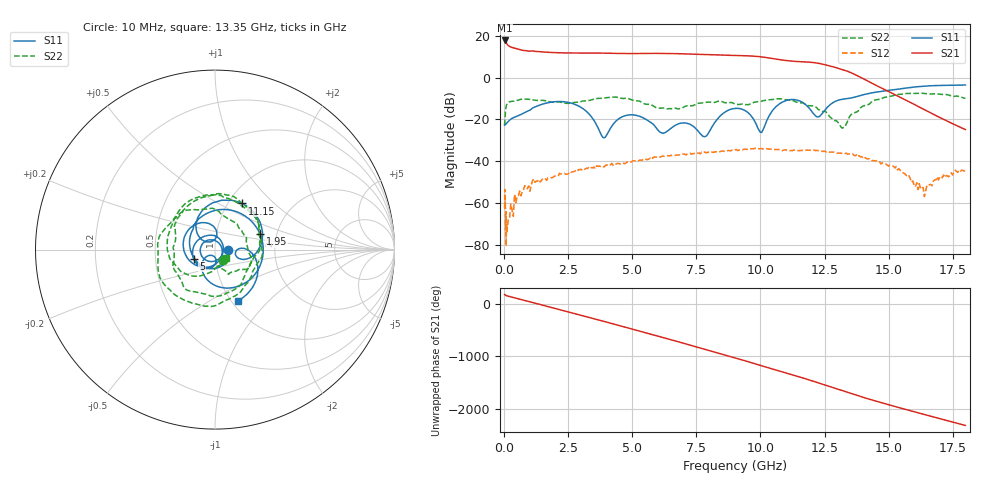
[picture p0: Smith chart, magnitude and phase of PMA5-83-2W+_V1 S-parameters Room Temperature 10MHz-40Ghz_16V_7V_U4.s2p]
!Mini-Circuits Laboratory
!S-Parameters
!Model: US-AMP-1
!Run / Lot / Date Code: N/A /  / N/A
!Fixture: ON TB-
!Network Analyzer: NFA N8975A;  Serial number: 74408
!Date: 12/1/2023 at 8:04:13 AM
!No.: Unit# 1 (#1)
!Tested with:
!Condition 5: Vdd = +16V; Vg2= +7V; Idd= 400mA
# Hz  S  dB  R  50
!Frequency  S11 dB  S11 Deg  S21 dB  S21 Deg  S12 dB  S12 Deg  S22 dB  S22 Deg
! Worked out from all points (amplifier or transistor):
!   368 points, 10 MHz to 18 GHz, reference 50 ohm
!   highest |S21| = 17.8 dB at 20 MHz (marker M1)
!   |S21| within 3 dB of that: start of sweep to 227.9 MHz
!   unconditionally stable (mu >= 1): start of sweep to end of sweep
!   at 2.7 GHz: K = 19.95, MAG = 12.4 dB, |S12| = -44.9 dB
!   at 8.85 GHz: K = 7.35, MAG = 11.2 dB, |S12| = -34.9 dB
!   at 18 GHz: K = 696.48, MAG = -21.8 dB, |S12| = -44.1 dB
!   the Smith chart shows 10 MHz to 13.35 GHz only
!   S11 on the Smith chart (normalised r, x): 10 MHz: 1.16, -0.00; 1.95 GHz: 1.64, +0.30; 5 GHz: 0.78, -0.08; 11.15 GHz: 1.16, +0.65; 13.35 GHz: 1.06, -0.68
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1e7  -22.66 -0.7  17.63 177.2  -62.51 -60.1  -22.82 -50.6
2e7  -22.63 -3.0  17.80 174.1  -53.47 -85.4  -20.60 -79.6
5e8  -18.40 -141.9  13.78 101.1  -56.65 48.0  -10.88 142.5
1.1e9  -14.51 124.0  12.77 26.0  -49.24 -43.3  -10.61 75.7
1.95e9  -11.51 18.7  11.99 -82.8  -47.13 -143.1  -11.70 2.6
2.55e9  -11.97 -46.9  11.82 -159.5  -44.93 141.9  -12.11 -33.3
3.05e9  -14.65 -98.3  11.81 135.8  -44.42 84.0  -11.21 -58.5
4.05e9  -26.22 -85.8  11.69 4.1  -41.94 -44.2  -9.50 -129.6
5e9  -17.77 -157.4  11.54 -121.0  -39.89 -164.4  -10.72 151.0
5.5e9  -19.72 142.0  11.59 172.6  -38.99 133.5  -12.57 106.8
6.05e9  -25.79 33.3  11.62 98.3  -38.02 62.1  -14.61 61.2
6.75e9  -22.33 -127.3  11.48 2.4  -36.93 -27.0  -14.86 15.8
7.4e9  -23.47 128.9  11.22 -86.8  -36.32 -114.5  -13.18 -40.5
8.15e9  -22.75 -79.8  10.95 170.0  -35.71 146.9  -11.90 -105.1
9.05e9  -14.67 152.5  10.67 43.7  -34.35 30.4  -12.72 -169.5
9.95e9  -25.32 94.0  10.07 -87.6  -34.02 -94.9  -11.31 141.1
1.05e10  -15.27 128.2  9.10 -168.2  -34.38 -172.3  -10.40 94.5
1.115e10  -10.52 59.8  8.00 99.5  -34.94 100.3  -10.76 39.1
1.205e10  -16.93 -20.3  7.24 -34.6  -34.75 -29.9  -13.47 -30.4
1.335e10  -10.06 -66.4  3.28 119.1  -36.12 124.0  -22.14 -39.1
1.505e10  -6.01 123.7  -6.91 -130.6  -41.85 -105.2  -8.95 -116.9
1.8e10  -3.51 177.3  -24.80 -159.8  -44.15 79.8  -9.87 57.0
